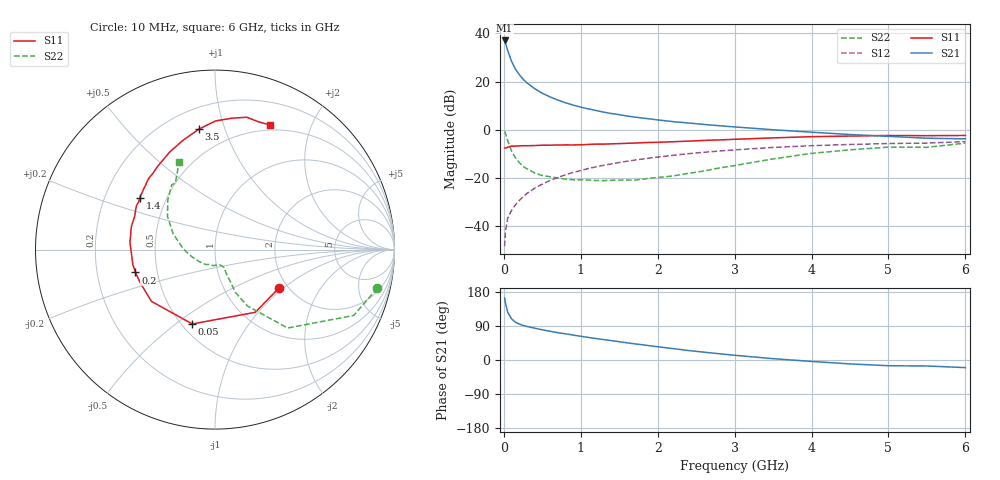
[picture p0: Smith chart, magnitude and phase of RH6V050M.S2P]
! SIEMENS Small Signal Semiconductors
! BFR106
! Si NPN RF Bipolar Junction Transistor in SOT23
! VCE = 6 V  IC = 50 mA
! Common Emitter S-Parameters:  August  1996
# GHz  S  MA  R  50
!  f  S11  S21  S12  S22
! GHz  MAG  ANG  MAG  ANG  MAG  ANG  MAG  ANG
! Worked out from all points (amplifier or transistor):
!   36 points, 10 MHz to 6 GHz, reference 50 ohm
!   highest |S21| = 37.1 dB at 10 MHz (marker M1)
!   |S21| within 3 dB of that: start of sweep to 39.47 MHz
!   unconditionally stable (mu >= 1): 248.6 MHz to 2.265 GHz
!   at 250 MHz: K = 1.00, MAG = 24.2 dB, |S12| = -27.9 dB
!   at 1.4 GHz: K = 1.06, MAG = 9.0 dB, |S12| = -14.2 dB
!   at 6 GHz: K = 0.98, MSG = 0.6 dB, |S12| = -5.0 dB
!   S11 on the Smith chart (normalised r, x): 10 MHz: 1.81, -0.93; 50 MHz: 0.56, -0.57; 200 MHz: 0.38, -0.12; 1.4 GHz: 0.35, +0.28; 3.5 GHz: 0.33, +0.82; 6 GHz: 0.44, +1.44
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0.01  0.4166 -30.5  71.58 163.9  0.0038 79.2  0.9294 -13.4
0.02  0.4151 -57.3  64.96 151.4  0.0075 75.0  0.8556 -25.4
0.05  0.4332 -107.0  44.31 126.1  0.0145 62.4  0.5954 -47.2
0.1  0.4566 -140.8  26.41 108.6  0.021 61.3  0.3619 -60.1
0.15  0.4561 -156.2  18.28 99.9  0.0273 63.7  0.2616 -64.6
0.2  0.4609 -164.0  14 95.0  0.0338 67.2  0.2089 -64.4
0.25  0.4656 -170.0  11.22 91.2  0.0402 68.5  0.1727 -64.6
0.3  0.4645 -173.6  9.421 88.5  0.0472 70.4  0.1541 -64.8
0.4  0.4687 179.9  7.138 84.0  0.0607 71.5  0.1262 -64.0
0.5  0.4757 175.0  5.729 79.7  0.0741 72.0  0.1116 -63.4
0.6  0.4763 171.1  4.799 75.9  0.088 71.3  0.1053 -64.6
0.7  0.481 166.8  4.142 72.2  0.1015 70.7  0.0996 -67.3
0.9  0.4828 160.2  3.251 65.8  0.1293 68.8  0.091 -71.1
1.1  0.4948 153.4  2.705 59.5  0.1562 66.5  0.09 -80.7
1.4  0.5094 145.3  2.167 51.1  0.1953 62.6  0.0888 -94.2
1.7  0.5273 137.2  1.831 42.6  0.2335 58.5  0.0896 -112.1
2.2  0.5631 124.7  1.471 30.1  0.2944 51.2  0.1093 -142.1
2.8  0.6134 110.9  1.211 16.5  0.3606 42.2  0.1603 -175.4
3.5  0.6763 97.8  0.998 3.5  0.4286 31.9  0.2478 159.7
4.5  0.7381 82.7  0.794 -10.3  0.4933 17.2  0.3819 133.6
5.5  0.7522 70.7  0.665 -15.8  0.5274 7.4  0.4306 120.9
6  0.7589 66.4  0.646 -20.1  0.5652 0.2  0.5271 112.3
